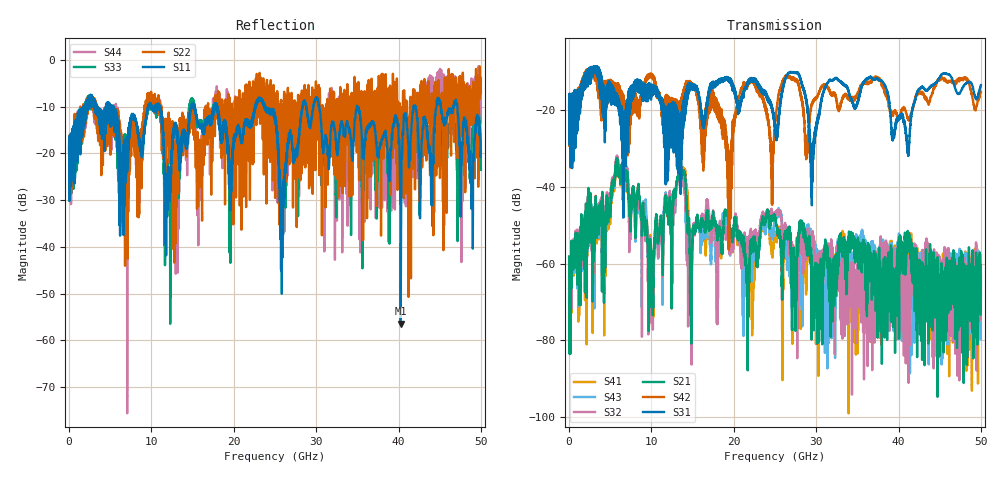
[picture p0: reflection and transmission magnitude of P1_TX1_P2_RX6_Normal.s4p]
!Keysight Technologies,N5225B,MY57041031,A.13.20.10
!Date: Friday, May 31, 2019 11:36:41
!Correction: S11(Full 4 Port(1,2,3,4))
!S12(Full 4 Port(1,2,3,4))
!S13(Full 4 Port(1,2,3,4))
!S14(Full 4 Port(1,2,3,4))
!S21(Full 4 Port(1,2,3,4))
!S22(Full 4 Port(1,2,3,4))
!S23(Full 4 Port(1,2,3,4))
!S24(Full 4 Port(1,2,3,4))
!S31(Full 4 Port(1,2,3,4))
!S32(Full 4 Port(1,2,3,4))
!S33(Full 4 Port(1,2,3,4))
!S34(Full 4 Port(1,2,3,4))
!S41(Full 4 Port(1,2,3,4))
!S42(Full 4 Port(1,2,3,4))
!S43(Full 4 Port(1,2,3,4))
!S44(Full 4 Port(1,2,3,4))
!S4P File: Measurements: <S11,S12,S13,S14>,
!<S21,S22,S23,S24>,
!<S31,S32,S33,S34>,
!<S41,S42,S43,S44>:
# Hz S  dB  R 50.0
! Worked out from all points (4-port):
!   5000 points, 10 MHz to 50 GHz, reference 50 ohm
!   strongest paths, dB at 10 MHz, 12.51 GHz, 25.01 GHz, 37.51 GHz, 50 GHz:
!     S31: -19.4, -29.3, -24.6, -11.8, -13.4
!     S42: -19.3, -16.9, -23.7, -11.6, -15.3
!     S21: -58.2, -48.0, -48.2, -61.7, -63.0
!     S32: -70.3, -56.5, -46.8, -66.2, -66.1
!     S43: -63.4, -61.2, -47.4, -65.0, -67.6
!     S41: -69.0, -49.9, -53.1, -70.7, -57.9
!   lowest |S11| = -56.4 dB at 40.27 GHz (marker M1), VSWR 1.00, Z = 49.9 + j0.0379 ohm
!   |S11| at or under -10 dB: 18.01 GHz to 22.61 GHz (4.596 GHz wide, 22.6 % of centre); 30.38 GHz to 34.94 GHz (4.563 GHz wide, 14 % of centre); 34.98 GHz to 41.82 GHz (6.84 GHz wide, 17.8 % of centre)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
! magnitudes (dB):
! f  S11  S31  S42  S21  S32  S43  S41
! 10 MHz  -20.0  -19.4  -19.3  -58.2  -70.3  -63.4  -69.0
! 5.85 GHz  -14.6  -17.6  -15.1  -32.5  -31.9  -32.1  -32.9
! 10.11 GHz  -9.9  -14.3  -11.7  -60.5  -64.7  -64.6  -60.8
! 13.39 GHz  -21.3  -24.9  -20.9  -36.7  -37.4  -37.3  -36.7
! 14.84 GHz  -10.2  -13.9  -13.2  -80.9  -63.2  -64.2  -67.7
! 40.27 GHz  -56.4  -21.3  -20.4  -58.4  -60.6  -61.5  -64.8
! 50 GHz  -19.7  -13.4  -15.3  -63.0  -66.1  -67.6  -57.9
